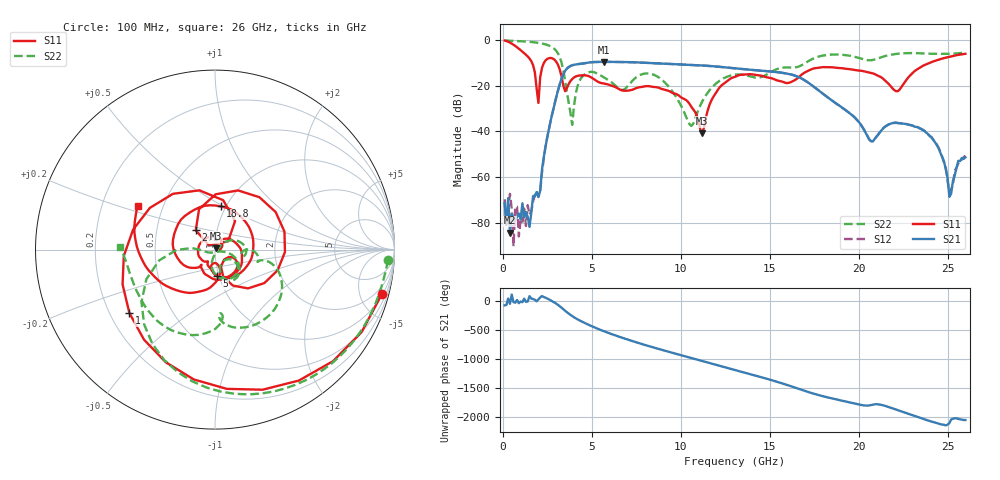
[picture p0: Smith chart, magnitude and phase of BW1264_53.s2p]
!Keysight Technologies,N5245B,MY57181159,A.13.60.06
!Date: Friday, December 18, 2020 23:54:52
!Correction: S11(Full 2 Port(1,2))
!S21(Full 2 Port(1,2))
!S12(Full 2 Port(1,2))
!S22(Full 2 Port(1,2))
!S2P File: Measurements: S11, S21, S12, S22:
# Hz S  dB  R 50
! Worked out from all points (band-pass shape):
!   260 points, 100 MHz to 26 GHz, reference 50 ohm
!   highest |S21| = -9.66 dB at 5.7 GHz (marker M1); lowest = -84.3 dB at 400 MHz (marker M2)
!   |S21| within 3 dB of the highest: 3.594 GHz to 13.24 GHz (9.648 GHz wide, 115 % of centre)
!   lowest |S11| = -40.9 dB at 11.2 GHz (marker M3), VSWR 1.02, Z = 50.6 + j0.673 ohm
!   |S11| at or under -10 dB: 1.638 GHz to 2.318 GHz (680.4 MHz wide, 34.4 % of centre); 3.031 GHz to 24.03 GHz (21 GHz wide, 155 % of centre)
!   |S22| runs from -37.7 to -0.3 dB; largest |S21 - S12| = 0.00057
!   S11 on the Smith chart (normalised r, x): 100 MHz: 1.11, -7.42; 1 GHz: 0.28, -0.31; 2.1 GHz: 0.79, +0.17; 5 GHz: 0.98, -0.29; 18.8 GHz: 0.94, +0.48; 26 GHz: 0.36, +0.23
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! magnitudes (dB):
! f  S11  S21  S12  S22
! 100 MHz  -0.3  -71.4  -69.7  -0.3
! 200 MHz  -0.6  -80.9  -80.7  -0.4
! 300 MHz  -0.9  -69.2  -75.2  -0.4
! 400 MHz  -1.2  -84.3  -67.3  -0.4
! 1 GHz  -4.5  -78.5  -78.9  -0.6
! 2 GHz  -27.6  -68.6  -68.8  -1.4
! 2.1 GHz  -16.4  -65.9  -66.1  -1.5
! 3.2 GHz  -13.0  -19.4  -19.4  -7.6
! 3.9 GHz  -17.1  -11.2  -11.1  -37.2
! 4.5 GHz  -15.5  -10.4  -10.4  -15.8
! 5 GHz  -16.6  -9.8  -9.8  -14.0
! 5.7 GHz  -19.1  -9.7  -9.7  -16.5
! 8.8 GHz  -21.1  -10.4  -10.4  -16.6
! 10.6 GHz  -29.3  -11.0  -11.0  -37.7
! 11.2 GHz  -40.9  -11.2  -11.2  -27.1
! 13.1 GHz  -16.1  -12.5  -12.6  -15.2
! 17.4 GHz  -12.7  -20.0  -20.0  -8.4
! 18.8 GHz  -12.3  -28.2  -28.2  -6.5
! 21.7 GHz  -19.4  -36.9  -36.9  -6.7
! 24.1 GHz  -9.8  -42.5  -42.8  -6.1
! 25.1 GHz  -7.4  -68.6  -67.0  -6.1
! 26 GHz  -6.1  -51.4  -50.7  -5.6
